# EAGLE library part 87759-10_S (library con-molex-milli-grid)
HEADER
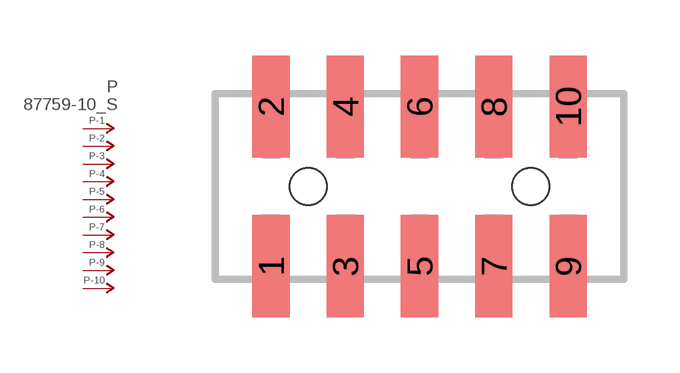
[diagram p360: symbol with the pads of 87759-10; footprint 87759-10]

Designator prefix P; gates -1=P-NV -2=P-N -3=P-N -4=P-N -5=P-N -6=P-N -7=P-N -8=P-N -9=P-N -10=P-N

## 87759-10_S  [87759-10]
1  -1:P  pas
2  -2:P  pas
3  -3:P  pas
4  -4:P  pas
5  -5:P  pas
6  -6:P  pas
7  -7:P  pas
8  -8:P  pas
9  -9:P  pas
10  -10:P  pas

## Footprint 87759-10 (pad centres in mm)
HEADER SMD Dual Row, Vertical
smd 1 x 2.75: 1 -4,-2.15; 2 -4,2.15; 3 -2,-2.15; 4 -2,2.15; 5 0,-2.15; 6 0,2.15; 7 2,-2.15; 8 2,2.15; 9 4,-2.15; 10 4,2.15
hole 1 at -3,0
hole 1 at 3,0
